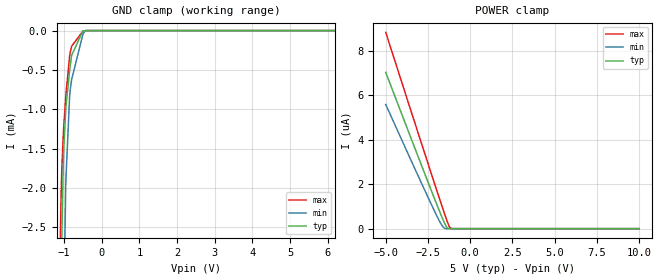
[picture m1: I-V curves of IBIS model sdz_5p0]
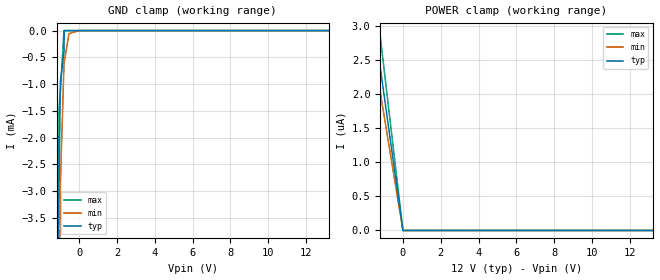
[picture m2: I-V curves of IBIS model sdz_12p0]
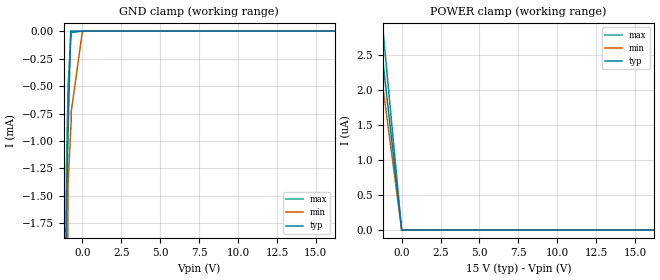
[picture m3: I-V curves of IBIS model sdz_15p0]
|Texas Instruments Incorporated
| Inductor Free Stereo(BTL) 10W Class-D Audio Amplifier with ultra low EMI
| and Auto Gain Limiter
| Marketing part#   Digital Voltage Range   Package-type   #pins
| TPA3140D2PWP   4.5V-16.5V   HTSSOP   28
| TPA3140D2PWPR   4.5V-16.5V   HTSSOP   28
[IBIS Ver]   4.1
[File name]   tpa3140d2.ibs
[File Rev]   1.0
[Date]   3/10/2015
[Source]
| Texas Instruments Incorporated.
| Analog-eLab Design Center, HPA
| 12500 TI Blvd
| Dallas, TX -75243
[Notes]   Revision History:
| Rev 1.0: 3/10/2015
| - Initial version of the model
| - Model generated from simulations in SPECTRE
| - Model matched to SPICE simulation
| - C_comp although listed in numerical order of value are
|   obtained from varying PVT conditions. For PVT conditions for
|   each specific value refer the buffer description under
|   respective [Model]. IBIS model user is responsible for using
|   appropriate C_comp to simulate for Signal Integrity.
[Disclaimer]
| This model is designed as an aid for customers of Texas Instruments.
| TI and its licensors and suppliers make no warranties, either expressed
| or implied, with respect to this  model, including the warranties of
| merchantability or fitness for a particular purpose. The model is
| provided solely on an "as is" basis. The entire risk as to its quality
| and performance is with the customer.
[Copyright]
(C) Copyright 2015 Texas Instruments Incorporated.All rights reserved.
|   TPA3140D2PWP
[Component]   TPA3140D2PWP
[Manufacturer]   TI
[Package]   |28 HTSSOP  -  PWP package
|   typ   min   max
R_pkg   0.08031   0.07956   0.08105
L_pkg   3.91881nH   3.74443nH   4.09319nH
C_pkg   0.65863pF   0.64256pF   0.67469pF
[Pin]  signal_name   model_name   R_pin   L_pin   C_pin
1   _SD   SDZ   0.08105   4.09319nH  0.67469pF
2   _FAULT   FAULTZ   0.07956   3.74443nH  0.64256pF
3   LINP   NC   0.06337   2.88658nH  0.51602pF
4   LINN   NC   0.05011   2.38821nH  0.49018pF
5   GAIN0   NC   0.04019   2.02497nH  0.45719pF
6   GAIN1   NC   0.03842   1.96451nH  0.44847pF
7   AVCC   POWER   0.04061   2.04349nH  0.44806pF
8   AGND   GND   0.03967   2.00969nH  0.44534pF
9   GVDD   POWER   0.03853   1.97183nH  0.44851pF
10   PLIMIT   NC   0.04002   2.01869nH  0.45397pF
11   RINN   NC   0.05011   2.38803nH  0.49058pF
12   RINP   NC   0.06337   2.88657nH  0.51635pF
13   NC   NC   0.07942   3.73975nH  0.63566pF
14   PBTL   NC   0.08269   4.15951nH  0.67446pF
15   PVCCR   POWER   0.04812   3.67297nH  0.74556pF
16   PVCCR   POWER   0.07783   3.66911nH  0.64704pF
17   BSPR   NC   0.07260   3.22359nH  0.55615pF
18   OUTPR   NC   0.03113   2.18232nH  0.56772pF
19   PGND   GND   0.02663   1.89161nH  0.52882pF
20   OUTNR   NC   0.02705   1.92104nH  0.52020pF
21   BSNR   NC   0.04954   2.35322nH  0.48154pF
22   BSNL   NC   0.04954   2.35322nH  0.48154pF
23   OUTNL   NC   0.02702   1.91633nH  0.51731pF
24   PGND   GND   0.02663   1.89156nH  0.52882pF
25   OUTPL   NC   0.03114   2.18257nH  0.56774pF
26   BSPL   NC   0.07261   3.22364nH  0.55609pF
27   PVCCL   POWER   0.07782   3.66852nH  0.64703pF
28   PVCCL   POWER   0.04807   3.66778nH  0.74326pF
|   Model Selectors
[Model Selector] SDZ
sdz_5p0   5.0V   digital Input
sdz_12p0   12.0V  digital Input
sdz_15p0   15.0V  digital Input
[Model Selector] FAULTZ
faultz_5p0   5.0V   digital  Open_drain
faultz_12p0   12.0V  digital  Open_drain
faultz_15p0   15.0V  digital  Open_drain
| Models and submodels in the file (6): sdz_5p0 (Input), sdz_12p0 (Input), sdz_15p0 (Input), faultz_5p0 (Open_drain), faultz_12p0 (Open_drain), faultz_15p0 (Open_drain)
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|   sdz_5p0 Model
[Model]   sdz_5p0
Model_type   Input
Vinl = 0.8
Vinh = 2
|   typ   min   max
|   (nom PVT)   (fast PVT)   (slow PVT)
C_comp   1.418e-13   1.266e-13   1.692e-13
| Where nom  PVT is Nominal Process, 5V, 27C
|   Fast PVT is Strong Process,  5.5V, -40C
|   Slow PVT is Weak Process,   4.5V, 125C
[Voltage Range]   5   4.5   5.5
|Junction Temperature
[Temperature Range]   27   125   -40
[Power Clamp Reference]   5   4.5   5.5
[GND Clamp Reference]   0   0   0
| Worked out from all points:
|   GND clamp passes 1 mA (typ) near -0.95 V on its own axis
[GND Clamp]
|   Voltage   I(typ)   I(min)   I(max)
-5V       -269.7mA   -266.6mA   -277.1mA
-1.106V   -4.373mA   -7.765mA   -2.84mA
-1.081V   -3.338mA   -6.512mA   -2.145mA
-1.06V    -2.639mA   -5.57mA    -1.769mA
-1.02V    -1.683mA   -3.914mA   -1.319mA
-1.008V   -1.504mA   -3.486mA   -1.223mA
-950mV    -966.8uA   -1.885mA   -808.4uA
-853mV    -511.3uA   -842.5uA   -323.4uA
-800mV    -315.8uA   -625.8uA   -199.6uA
-500mV    -4.86uA    -48.01uA   -8.145uA
-437mV    -3.329uA   0A         -2.298uA
10V       0A         0A         0A
[POWER Clamp]
|   Voltage   I(typ)   I(min)   I(max)
-5V       7.038uA    5.592uA    8.841uA
-2.566V   2.23uA     1.524uA    3.091uA
-1.814V   782nA      334.5nA    1.341uA
-1.605V   399.1nA    72.98nA    864.7nA
-1.425V   108.2nA    0A         466nA
-1.3V     0A         0A         208.4nA
-1.188V   0A         0A         38.01nA
-1.04V    0A         0A         0A
10V       0A         0A         0A
|   sdz_12p0 Model
[Model]   sdz_12p0
Model_type   Input
Vinl = 0.8
Vinh = 2
|   typ   min   max
|   (nom PVT)   (fast PVT)   (slow PVT)
C_comp   1.418e-13   1.266e-13   1.692e-13
| Where nom  PVT is Nominal Process, 12V, 27C
|   Fast PVT is Strong Process,  13.2V, -40C
|   Slow PVT is Weak Process,   10.8V, 125C
[Voltage Range]   12   10.8   13.2
|Junction Temperature
[Temperature Range]   27   125   -40
[Power Clamp Reference]   12   10.8   13.2
[GND Clamp Reference]   0   0   0
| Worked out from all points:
|   GND clamp passes 1 mA (typ) near -1.00 V on its own axis
[GND Clamp]
|   Voltage   I(typ)   I(min)   I(max)
-12V      -947.7mA   -759.1mA   -1.163A
-1.15V    -6.287mA   -9.704mA   -4.494mA
-1.124V   -5.013mA   -8.379mA   -3.417mA
-1.116V   -4.184mA   -7.955mA   -2.901mA
-1.084V   -3.328mA   -6.365mA   -1.793mA
-1.056V   -2.644mA   -5.117mA   -1.399mA
-996mV    -948.5uA   -2.876mA   -1.14mA
-806.4mV  -402.2uA   -631.4uA   0A
-792mV    0A         -586.5uA   0A
-541.2mV  0A         -56.57uA   0A
-12mV     0A         0A         0A
24V       0A         0A         0A
[POWER Clamp]
|   Voltage   I(typ)   I(min)   I(max)
-12V      23.93uA    20.35uA    28.53uA
-2.16V    4.301uA    3.652uA    5.129uA
-1.692V   3.369uA    2.86uA     4.017uA
-1.664V   3.314uA    2.813uA    3.951uA
-1.2V     2.389uA    2.027uA    2.848uA
-1.2mV    0A         0A         0A
24V       0A         0A         0A
|   sdz_15p0 Model
[Model]   sdz_15p0
Model_type   Input
Vinl = 0.8
Vinh = 2
|   typ   min   max
|   (nom PVT)   (fast PVT)   (slow PVT)
C_comp   1.418e-13   1.266e-13   1.692e-13
| Where nom  PVT is Nominal Process, 15V, 27C
|   Fast PVT is Strong Process,  16.5V, -40C
|   Slow PVT is Weak Process,   13.5V, 125C
[Voltage Range]   15   13.5   16.5
|Junction Temperature
[Temperature Range]   27   125   -40
[Power Clamp Reference]   15   13.5   16.5
[GND Clamp Reference]   0   0   0
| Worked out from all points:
|   GND clamp passes 1 mA (typ) near -0.94 V on its own axis
[GND Clamp]
|   Voltage   I(typ)   I(min)   I(max)
-15V      -1.441A    -1.142A    -1.678A
-1.122V   -4.46mA    -7.698mA   -2.941mA
-1.028V   -1.651mA   -4.28mA    -1.23mA
-925.5mV  -912.3uA   -1.392mA   -502.6uA
-757.5mV  0A         -901.9uA   -75.43uA
-730.5mV  0A         -829.6uA   -51.59uA
-727.5mV  0A         -737.5uA   -14.75uA
-1.5mV    0A         0A         0A
30V       0A         0A         0A
[POWER Clamp]
|   Voltage   I(typ)   I(min)   I(max)
-15V      29.94uA    25.47uA    35.69uA
-2.107V   4.202uA    3.57uA     5.008uA
-1.5V     2.991uA    2.54uA     3.563uA
-1.392V   2.775uA    2.357uA    3.306uA
-1.298V   2.587uA    2.197uA    3.081uA
-1.11V    2.213uA    1.879uA    2.636uA
-1.5mV    0A         0A         0A
30V       0A         0A         0A
